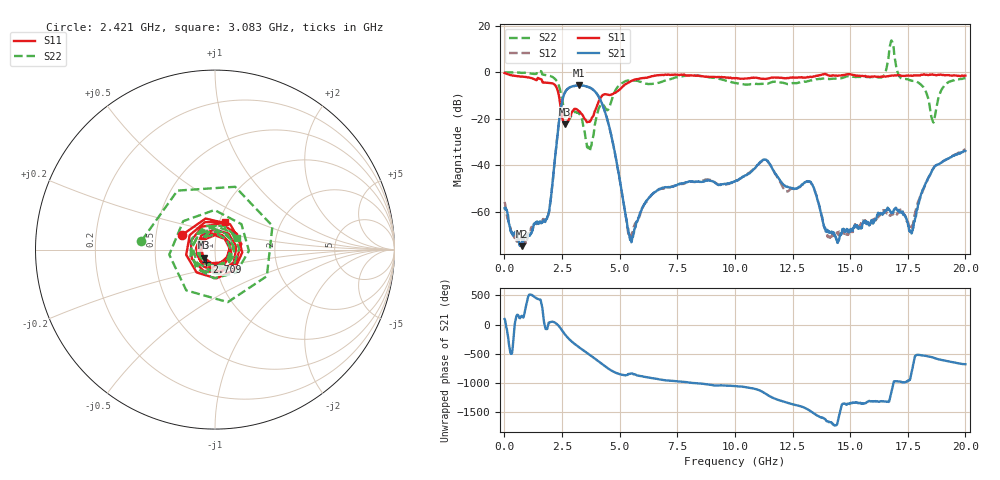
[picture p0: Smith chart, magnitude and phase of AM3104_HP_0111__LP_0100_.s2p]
!Created with skrf (http://scikit-rf.org).
# Hz S RI R 50.0
!freq ReS11 ImS11 ReS21 ImS21 ReS12 ImS12 ReS22 ImS22
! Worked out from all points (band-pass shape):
!   1601 points, 10 MHz to 20 GHz, reference 50 ohm
!   highest |S21| = -5.66 dB at 3.246 GHz (marker M1); lowest = -74.7 dB at 759.6 MHz (marker M2)
!   |S21| within 3 dB of the highest: 2.629 GHz to 3.966 GHz (1.337 GHz wide, 40.5 % of centre)
!   lowest |S11| = -22.2 dB at 2.609 GHz (marker M3), VSWR 1.17, Z = 43.8 - j3.89 ohm
!   |S11| at or under -10 dB: 2.365 GHz to 4.245 GHz (1.88 GHz wide, 56.9 % of centre)
!   |S22| runs from -34.0 to 13.6 dB; largest |S21 - S12| = 0.028
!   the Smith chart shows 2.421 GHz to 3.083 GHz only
!   S11 on the Smith chart (normalised r, x): 2.421 GHz: 0.68, +0.12; 2.709 GHz: 0.90, -0.13; 3.083 GHz: 1.07, +0.34
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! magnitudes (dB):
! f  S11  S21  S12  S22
! 10 MHz  -0.4  -58.4  -55.7  0.0
! 759.6 MHz  -1.9  -74.7  -71.3  -0.3
! 1.872 GHz  -4.6  -62.0  -62.1  -1.3
! 2.421 GHz  -13.9  -17.2  -17.3  -7.7
! 2.609 GHz  -22.2  -9.1  -9.1  -17.4
! 2.709 GHz  -21.4  -7.5  -7.5  -20.8
! 3.083 GHz  -15.7  -5.8  -5.8  -17.0
! 3.246 GHz  -16.9  -5.7  -5.8  -18.0
! 3.346 GHz  -17.9  -5.7  -5.8  -19.3
! 3.683 GHz  -21.3  -6.5  -6.6  -33.9
! 4.37 GHz  -9.4  -17.2  -17.2  -15.3
! 5.482 GHz  -3.9  -71.3  -70.0  -3.6
! 6.682 GHz  -1.2  -50.5  -50.4  -4.6
! 10.01 GHz  -2.7  -46.9  -47.0  -4.6
! 11.3 GHz  -2.9  -37.5  -37.8  -5.0
! 12.22 GHz  -2.6  -49.1  -51.3  -4.9
! 13.34 GHz  -2.1  -48.1  -48.1  -3.5
! 14.43 GHz  -1.5  -71.9  -69.2  -2.8
! 16.68 GHz  -1.6  -59.0  -61.0  7.2
! 17.65 GHz  -1.5  -68.8  -66.7  -3.6
! 18.59 GHz  -1.0  -41.7  -41.7  -21.1
! 20 GHz  -1.5  -33.8  -33.1  -2.5
